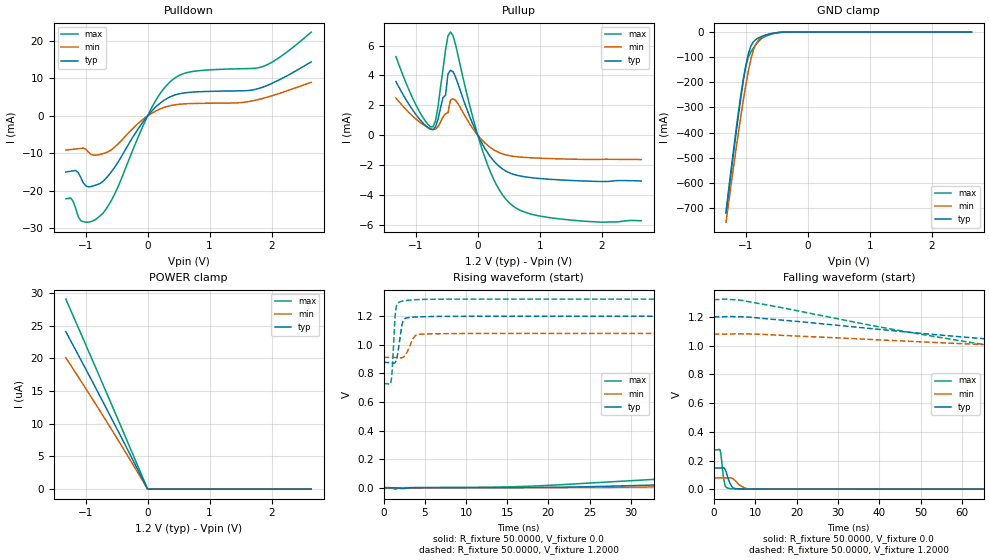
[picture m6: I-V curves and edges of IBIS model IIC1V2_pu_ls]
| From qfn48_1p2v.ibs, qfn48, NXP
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[Model] IIC1V2_pu_ls
|   Model IIC1V2_pu_ls
| This model was characterised for following simulation conditions:
| External (pad) voltage:
|   - Typ: 1.2V,   - Min: 1.08V,   - Max: 1.32V
| Library cells for typ/min/max conditions are connected as defined below:
|  IO - External Pad
|  A - Core Input
|  EN - Output Buffer Enable
|  BOOST - vdde
|  EGP - vdd
|  EHS - gnd
|  ENZI - vdd
|  EPD - gnd
|  EPUN - gnd
|  ZI - NC
|  ZIF - NC
|  gnd - gnd
|  gnde - gnde
|  vdd - vdd
|  vdde - vdde
| All other pins connected to ground
Model_type I/O
Polarity   Non-Inverting
Enable   Active-Low
Vinl =   0.5400V
Vinh =   1.2600V
Vmeas =  0.9000V
Cref =   0.0F
Rref =   1.0000k
Vref =   0.0V
C_comp   3.6132pF   3.4729pF   3.7394pF
|C_comp_pullup   0.9302pF   0.8892pF   0.9447pF
|C_comp_pulldown   2.3308pF   2.4848pF   2.1849pF
[Model Spec]
| variable   typ   min   max
Vinh   0.3600V   0.3240V   0.3960V
Vinl   0.8400V   0.7560V   0.9240V
Vmeas   0.6000V   0.5400V   0.6600V
[Temperature Range]   25.0000   0.1250k   -40.0000
[Voltage Range]   1.2000V   1.0800V   1.3200V
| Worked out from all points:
|   slope of the pulldown table from 0 to 0.18 V, typ, clamps not added: 58.3 ohm
|   slope of the pullup table from 0 to 0.18 V, typ, clamps not added: 138 ohm
|   GND clamp passes 1 mA (typ) near -0.45 V on its own axis
|   rising waveform, R_fixture 50.0000, V_fixture 0.0: 20-80 % time 73.4ns typ, 82.8ns min, 61.8ns max; typ from 0.001 V to 0.147 V
|   rising waveform, R_fixture 50.0000, V_fixture 1.2000: 20-80 % time 494ps typ, 787ps min, 328ps max; typ from 0.877 V to 1.2 V
|   falling waveform, R_fixture 50.0000, V_fixture 0.0: 20-80 % time 1.13ns typ, 1.91ns min, 702ps max; typ from 0.147 V to 0.001 V
|   falling waveform, R_fixture 50.0000, V_fixture 1.2000: 20-80 % time 83.3ns typ, 98.9ns min, 62.7ns max; typ from 1.2 V to 0.877 V
[Pulldown]
|Voltage   I(typ)   I(min)   I(max)
-1.32V    -14.96mA   -9.099mA   -22.09mA
-1.24V    -14.75mA   -8.982mA   -21.89mA
-1.16V    -14.56mA   -8.83mA    -24.7mA
-1.04V    -17.82mA   -8.609mA   -28.21mA
-920mV    -18.88mA   -10.21mA   -28.21mA
-720mV    -17.44mA   -10.07mA   -25.94mA
-520mV    -13.41mA   -8.157mA   -20.44mA
80mV      1.521mA    840uA      2.628mA
440mV     5.569mA    2.951mA    10.1mA
760mV     6.377mA    3.307mA    11.92mA
1.84V     7.555mA    4.581mA    13.06mA
2.64V     14.41mA    8.944mA    22.34mA
[Pullup]
|Voltage   I(typ)   I(min)   I(max)
-1.32V    3.586mA    2.483mA    5.256mA
-960mV    1.175mA    947.9uA    1.725mA
-720mV    361.7uA    375.8uA    554.6uA
-640mV    1.072mA    568.6uA    1.915mA
-520mV    2.67mA     1.432mA    5.707mA
-480mV    4.094mA    1.5mA      6.648mA
-440mV    4.342mA    2.345mA    6.901mA
120mV     -924.8uA   -536.9uA   -1.554mA
360mV     -2.143mA   -1.197mA   -3.751mA
600mV     -2.653mA   -1.434mA   -4.838mA
1.4V      -3.016mA   -1.6mA     -5.648mA
2.64V     -3.069mA   -1.636mA   -5.736mA
[GND_clamp]
|Voltage   I(typ)   I(min)   I(max)
-1.32V    -720.7mA   -756.5mA   -713.8mA
-1.12V    -330.9mA   -399.5mA   -316.8mA
-1.04V    -192.5mA   -269.2mA   -184.5mA
-1V       -133.6mA   -209.3mA   -133.5mA
-960mV    -86.76mA   -154.8mA   -99.49mA
-920mV    -55.71mA   -108.2mA   -79.05mA
-880mV    -39.04mA   -72.36mA   -63.74mA
-840mV    -29.93mA   -48.01mA   -50.29mA
-760mV    -18.95mA   -23.41mA   -28.35mA
-640mV    -9.243mA   -8.645mA   -12.76mA
-400mV    -357.8uA   -419.3uA   -472.1uA
2.64V     0A         0A         0A
[POWER_clamp]
|Voltage   I(typ)   I(min)   I(max)
-1.32V    24.09uA    20.1uA     29.06uA
-640mV    11.88uA    10.01uA    14.23uA
0V        86.89pA    4.342nA    7.851pA
2.64V     0A         0A         0A
[Ramp]
| variable   typ   min   max
dV/dt_r  87.9871m/73.3841n   46.5407m/82.8685n   0.1640/61.7493n
dV/dt_f  0.1938/83.2885n   0.1006/98.8793n   0.3549/62.7048n
R_load = 50.0000
[Rising Waveform]
R_fixture= 50.0000
V_fixture= 0.0
V_fixture_min= 0.0
V_fixture_max= 0.0
|time   V(typ)   V(min)   V(max)
0s        557uV      548.4uV    536.1uV
1.445ns   -97.64uV   674uV      -9.695mV
2.431ns   -5.508mV   58.35uV    850.8uV
18.09ns   2.301mV    1.167mV    11.72mV
57.66ns   56.38mV    23.16mV    136.8mV
96.9ns    103.5mV    48.06mV    225.4mV
116.4ns   120mV      57.32mV    250.3mV
148.6ns   136.5mV    67.9mV     266.9mV
263.6ns   146.8mV    77.41mV    273.6mV
1us       147.2mV    78.12mV    273.9mV
[Rising Waveform]
R_fixture= 50.0000
V_fixture= 1.2000
V_fixture_min= 1.0800
V_fixture_max= 1.3200
|time   V(typ)   V(min)   V(max)
0s        876.9mV    912.3mV    728.5mV
903ps     875.1mV    912.6mV    744mV
1.063ns   872.9mV    912.5mV    844.7mV
1.395ns   875.8mV    911.4mV    1.204V
1.672ns   926.8mV    910mV      1.287V
2.229ns   1.141V     909.8mV    1.305V
2.529ns   1.181V     920.7mV    1.308V
3.867ns   1.194V     1.065V     1.316V
6.412ns   1.199V     1.077V     1.319V
1us       1.2V       1.08V      1.32V
[Falling Waveform]
R_fixture= 50.0000
V_fixture= 0.0
V_fixture_min= 0.0
V_fixture_max= 0.0
|time   V(typ)   V(min)   V(max)
0s        147.2mV    78.15mV    273.9mV
1.54ns    147.3mV    78.15mV    269.7mV
1.726ns   148mV      78.13mV    240.5mV
2.308ns   149.7mV    78.08mV    91.29mV
2.899ns   127.6mV    78.64mV    16.54mV
4.265ns   24.08mV    77.86mV    3.471mV
5.645ns   3.271mV    45.32mV    2.175mV
7.94ns    1.557mV    4.922mV    1.82mV
12.73ns   1.252mV    1.086mV    1.264mV
1us       557uV      548.5uV    536.1uV
[Falling Waveform]
R_fixture= 50.0000
V_fixture= 1.2000
V_fixture_min= 1.0800
V_fixture_max= 1.3200
|time   V(typ)   V(min)   V(max)
0s        1.2V       1.08V      1.32V
6.537ns   1.2V       1.081V     1.316V
44.28ns   1.101V     1.034V     1.107V
72.21ns   1.032V     998.7mV    972.4mV
96.38ns   982.1mV    974.3mV    814.1mV
115.3ns   941.3mV    958.9mV    763mV
137.4ns   904.5mV    944mV      741.5mV
177ns     882.8mV    925.8mV    731.5mV
267.8ns   877.7mV    914.1mV    729mV
1us       877mV      912.4mV    728.6mV
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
